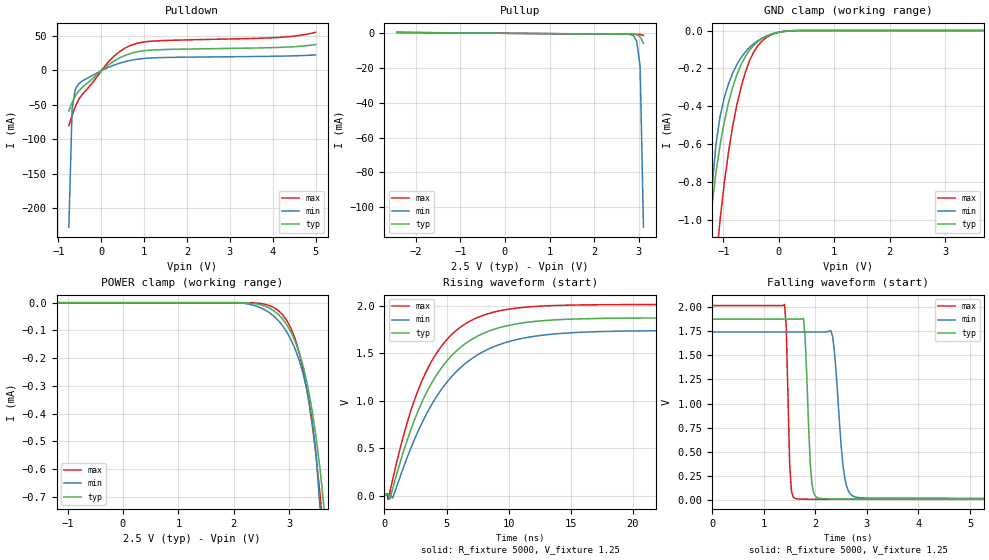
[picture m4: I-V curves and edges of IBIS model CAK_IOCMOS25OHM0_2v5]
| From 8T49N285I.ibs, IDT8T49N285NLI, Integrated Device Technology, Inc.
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[Model] CAK_IOCMOS25OHM0_2v5
Model_type   I/O
Polarity   Non-Inverting
|   typ   min   max
C_comp   2pF   1.5pF   2.5pF
|Input
Vinl = 0.7V
Vinh = 1.7V
|Output
Vmeas = 1.25V
Rref = 5000
Cref = 0
Vref = 1.25V
|   typ   min   max
[Voltage range]   2.5V   2.375V   2.625V
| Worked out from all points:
|   slope of the pulldown table from 0 to 0.375 V, typ, clamps not added: 22 ohm
|   slope of the pullup table from 0 to 0.375 V, typ, clamps not added: 5.02 kohm
|   GND clamp passes 1 mA (typ) near -1.23 V on its own axis
|   rising waveform, R_fixture 5000, V_fixture 1.25: 20-80 % time 4.26ns typ, 4.83ns min, 3.73ns max; typ from 0.013 V to 1.87 V
|   falling waveform, R_fixture 5000, V_fixture 1.25: 20-80 % time 84.6ps typ, 144ps min, 56.5ps max; typ from 1.87 V to 0.013 V
[GND_clamp]
|Voltage   I (typ)   I (min)   I (max)
-2.5V     -691.1mA   -685.3mA   -729.1mA
-1.288V   -1.205mA   -1.292mA   -1.977mA
-1.212V   -940.6uA   -855.1uA   -1.546mA
-1.136V   -752.2uA   -603.2uA   -1.235mA
-1.061V   -604.7uA   -452.9uA   -998.8uA
-984.8mV  -483.1uA   -354.8uA   -805.7uA
-833.3mV  -299.1uA   -225uA     -505.1uA
-681.8mV  -180.2uA   -143.3uA   -299.4uA
-454.5mV  -78.73uA   -69.94uA   -114.3uA
-227.3mV  -29.72uA   -30.67uA   -37.24uA
303mV     -612.1nA   -216.8nA   -565.8nA
5V        291.2pA    4.015nA    197.1pA
[Power_clamp]
|Voltage   I (typ)   I (min)   I (max)
-2.5V     291.2pA    3.748nA    294pA
2.121V    -116.9nA   -750.3nA   -7.756nA
2.727V    -29.72uA   -49.2uA    -17.96uA
2.879V    -58.11uA   -82.22uA   -42.91uA
3.03V     -104.8uA   -132.2uA   -90.92uA
3.182V    -180.2uA   -207.9uA   -180.2uA
3.258V    -233uA     -260.6uA   -247.2uA
3.409V    -381.8uA   -414.4uA   -428.8uA
3.485V    -483.1uA   -542.1uA   -550.4uA
3.561V    -604.7uA   -750.9uA   -696.6uA
3.636V    -752.2uA   -1.111mA   -869.5uA
5V        -691.1mA   -826.4mA   -494.6mA
[Pulldown]
|Voltage   I (typ)   I (min)   I (max)
|Note, modeling breaks down at 250mA and above.  This is well beyond the functional   |
|operating range of the device.  Should this scenario occur, catastrophic failure and   |
|possible damage to the device and/or board is of higher concern than the I-V curve   |
|behavior.  The IBIS checker will flag currents in excess of 10A with warnings.  Lines   |
|with currents in excess of 0.35 A have been commented out.  The points still remain|
|available to the user if the user desires to use them.   |
|-2.424240e+00   -1.111781e+01   -8.926054e+00   -1.358500e+01
|-2.348480e+00   -1.065838e+01   -8.583187e+00   -1.299865e+01
|-2.272730e+00   -1.019498e+01   -8.238442e+00   -1.240493e+01
|-2.196970e+00   -9.725751e+00   -7.891236e+00   -1.179892e+01
|-2.121210e+00   -9.247086e+00   -7.540665e+00   -1.116710e+01
|-2.045450e+00   -8.754719e+00   -7.185112e+00   -1.048970e+01
|-1.969700e+00   -8.235925e+00   -6.824277e+00   -9.780494e+00
|-1.893940e+00   -7.693129e+00   -6.454437e+00   -9.063475e+00
|-1.818180e+00   -7.137365e+00   -6.069098e+00   -8.346379e+00
|-1.742420e+00   -6.576462e+00   -5.669756e+00   -7.626942e+00
|-1.666670e+00   -6.013829e+00   -5.259747e+00   -6.908942e+00
|-1.590910e+00   -5.449978e+00   -4.843332e+00   -6.187923e+00
|-1.515150e+00   -4.885104e+00   -4.423353e+00   -5.465388e+00
|-1.439390e+00   -4.319487e+00   -4.001503e+00   -4.741877e+00
|-1.363640e+00   -3.753428e+00   -3.578693e+00   -4.017994e+00
|-1.287880e+00   -3.187195e+00   -3.155398e+00   -3.293993e+00
|-1.212120e+00   -2.620929e+00   -2.731885e+00   -2.569934e+00
|-1.136360e+00   -2.054718e+00   -2.308297e+00   -1.845855e+00
|-1.060610e+00   -1.488615e+00   -1.884737e+00   -1.121821e+00
|-9.848480e-01   -9.226489e-01   -1.461275e+00   -4.033103e-01
|-9.090910e-01   -3.622732e-01   -1.038018e+00   -1.161645e-01
|-8.333330e-01   -9.093424e-02   -6.150880e-01   -9.366890e-02
-757.6mV  -58.63mA   -227.5mA   -80.07mA
-681.8mV  -46.41mA   -55.85mA   -65.22mA
-606.1mV  -36.96mA   -27.07mA   -52.15mA
-530.3mV  -30mA      -19.55mA   -42.3mA
-454.5mV  -25.12mA   -15.8mA    -35.64mA
151.5mV   7.471mA    4.17mA     11.49mA
303mV     13.93mA    7.984mA    21.09mA
530.3mV   21.2mA     12.43mA    31.59mA
833.3mV   27.06mA    16.27mA    39.48mA
1.439V    30.33mA    18.78mA    43.38mA
4.167V    33.55mA    20.79mA    48.14mA
5V        37.61mA    22.61mA    55.4mA
[Pullup]
|Voltage   I (typ)   I (min)   I (max)
|Note, modeling breaks down at 250mA and above.  This is well beyond the functional   |
|operating range of the device.  Should this scenario occur, catastrophic failure and   |
|possible damage to the device and/or board is of higher concern than the I-V curve   |
|behavior.  The IBIS checker will flag currents in excess of 10A with warnings.  Lines   |
|with currents in excess of 0.35 A have been commented out.  The points still remain|
|available to the user if the user desires to use them.   |
-2.424V   482.9uA    423.1uA    557.9uA
2.727V    -513.6uA   -454.6uA   -609.7uA
2.879V    -541.1uA   -1.384mA   -619.7uA
2.955V    -754.7uA   -4.602mA   -620uA
3.03V     -1.986mA   -19.1mA    -670.4uA
3.106V    -5.706mA   -111.6mA   -1.261mA
|3.181820e+00   -1.238503e-02   -4.425551e-01   -4.339563e-03
|3.257580e+00   -2.230034e-02   -8.640044e-01   -1.166361e-02
|3.333330e+00   -5.275444e-02   -1.285923e+00   -2.253655e-02
|3.409090e+00   -3.224602e-01   -1.708196e+00   -3.494451e-02
|3.484850e+00   -8.813719e-01   -2.130688e+00   -4.653240e-02
|3.560610e+00   -1.446045e+00   -2.553319e+00   -9.388932e-02
|3.636360e+00   -2.011008e+00   -2.975989e+00   -5.959575e-01
|3.712120e+00   -2.576219e+00   -3.398581e+00   -1.318695e+00
|3.787880e+00   -3.141635e+00   -3.820865e+00   -2.041717e+00
|3.863640e+00   -3.707138e+00   -4.242452e+00   -2.764949e+00
|3.939390e+00   -4.272567e+00   -4.662614e+00   -3.488298e+00
|4.015150e+00   -4.837644e+00   -5.079986e+00   -4.211711e+00
|4.090910e+00   -5.402068e+00   -5.492135e+00   -4.935064e+00
|4.166670e+00   -5.965529e+00   -5.895342e+00   -5.657944e+00
|4.242420e+00   -6.527832e+00   -6.285540e+00   -6.379711e+00
|4.318180e+00   -7.088445e+00   -6.659737e+00   -7.099889e+00
|4.393940e+00   -7.643969e+00   -7.022868e+00   -7.817176e+00
|4.469700e+00   -8.186565e+00   -7.379891e+00   -8.531441e+00
|4.545450e+00   -8.705189e+00   -7.731628e+00   -9.253130e+00
|4.621210e+00   -9.197396e+00   -8.079611e+00   -9.969121e+00
|4.696970e+00   -9.675941e+00   -8.424863e+00   -1.067013e+01
|4.772730e+00   -1.014508e+01   -8.768094e+00   -1.133134e+01
|4.848480e+00   -1.060838e+01   -9.109740e+00   -1.195139e+01
|4.924240e+00   -1.106771e+01   -9.450169e+00   -1.255228e+01
|5.000000e+00   -1.152431e+01   -9.789506e+00   -1.314302e+01
[Ramp]
|   typ   min   max
dV/dt_r   1.143/4.278n   1.056/4.845n   1.231/3.738n
dV/dt_f   1.12/0.084n   1.04/0.144n   1.209/0.056n
R_load =   5000
[Rising Waveform]
R_fixture = 5000
V_fixture = 1.25   |Vcc_typ
V_fixture_min = 1.1875 |Vcc_min
V_fixture_max = 1.3125 |Vcc_max
C_fixture = 0.0p
| Time   typ   min   max
0s        12.95mV    19.9mV     9.777mV
300ps     14.4mV     19.85mV    -37.14mV
433.3ps   -32.86mV   21.11mV    35.92mV
666.7ps   77.13mV    -20.48mV   173.6mV
2.033ns   662.6mV    471mV      857.2mV
3.433ns   1.098V     873.5mV    1.327V
5.033ns   1.421V     1.197V     1.646V
7.033ns   1.647V     1.444V     1.849V
13.37ns   1.85V      1.7V       2.002V
30ns      1.874V     1.741V     2.015V
[Falling Waveform]
R_fixture = 5000
V_fixture = 1.25   |Vcc_typ
V_fixture_min = 1.1875 |Vcc_min
V_fixture_max = 1.3125 |Vcc_max
C_fixture = 0.0p
| Time   typ   min   max
0s        1.874V     1.741V     2.015V
1.4ns     1.874V     1.741V     2.025V
1.5ns     1.874V     1.741V     376.8mV
1.633ns   1.874V     1.741V     14.69mV
1.767ns   1.881V     1.741V     11.07mV
1.933ns   167.4mV    1.741V     10.44mV
2.1ns     18.17mV    1.741V     10.21mV
2.333ns   14.24mV    1.695V     10.06mV
2.833ns   13.42mV    27.99mV    9.917mV
30ns      12.96mV    19.91mV    9.781mV
